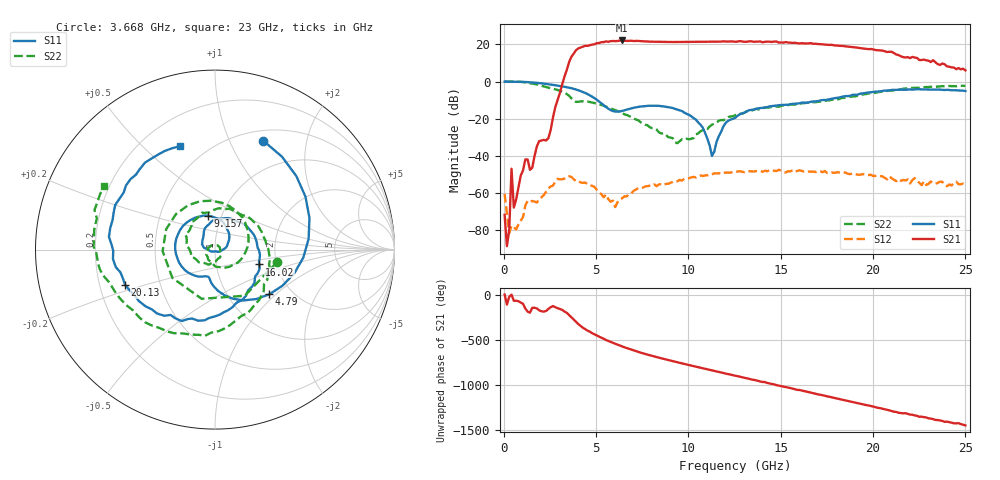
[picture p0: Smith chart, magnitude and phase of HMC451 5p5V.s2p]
!Hittite Microwave Corporation
!20 Alpha Road
!Chelmsford, MA 01824
!Tel: 978-250-3343
!Fax: 978-250-3373
!Device: HMC451, 5-20 GHz, Driver Amplifier Die
!Misc: Vcc = 5.5V, room. Die measured in housing that includes two K connectors, not de-embedded.
# MHZ S MA R 50
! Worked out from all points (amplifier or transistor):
!   201 points, 50 MHz to 25 GHz, reference 50 ohm
!   highest |S21| = 22.1 dB at 6.412 GHz (marker M1)
!   |S21| within 3 dB of that: 4.382 GHz to 18.4 GHz (14.02 GHz wide, 123 % of centre)
!   unconditionally stable (mu >= 1): start of sweep to end of sweep
!   at 4.167 GHz: K = 20.07, MAG = 20.3 dB, |S12| = -54.3 dB
!   at 12.53 GHz: K = 10.97, MAG = 21.5 dB, |S12| = -48.4 dB
!   at 25 GHz: K = 41.70, MAG = 11.5 dB, |S12| = -55.3 dB
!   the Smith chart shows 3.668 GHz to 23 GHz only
!   S11 on the Smith chart (normalised r, x): 3.668 GHz: 0.62, +1.34; 4.79 GHz: 1.54, -0.91; 9.157 GHz: 0.86, +0.34; 16.02 GHz: 1.63, -0.29; 20.13 GHz: 0.31, -0.17; 23 GHz: 0.36, +0.66
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50  0.997 -3.6  0.0002606 7.4  0.0009547 8.9  0.994 -3.9
3168.75  0.743 112.1  0.846 -162.6  0.002345 96.6  0.537 98.1
3667.75  0.664 66.2  4.674 114.0  0.002701 56.2  0.354 -11.0
3917.25  0.611 42.2  6.99 64.6  0.002066 31.6  0.284 -105.1
4291.5  0.525 6.5  8.704 -1.1  0.001883 19.2  0.295 157.3
4790.5  0.392 -39.4  9.864 -61.4  0.001564 5.8  0.273 94.1
5414.25  0.232 -85.4  11.52 -122.5  0.0007724 -4.3  0.224 40.7
5913.25  0.161 -101.5  12.33 -168.3  0.000627 14.8  0.181 3.8
6412.25  0.162 -112.5  12.76 151.7  0.0007245 51.9  0.145 -30.3
7285.5  0.208 -153.2  12.39 91.6  0.001365 42.7  0.091 -90.8
8408.25  0.222 143.8  11.68 26.9  0.00172 27.3  0.043 -165.6
9156.75  0.194 101.8  11.58 -11.5  0.002019 22.2  0.03 125.5
10778.5  0.058 8.4  11.76 -90.1  0.002875 3.7  0.049 -52.4
12525  0.105 126.8  11.77 -172.8  0.003784 -28.8  0.123 -157.3
14396.25  0.214 42.2  11.81 100.7  0.004109 -67.7  0.201 119.6
16018  0.261 -18.5  10.62 28.6  0.004087 -95.8  0.25 49.1
16766.5  0.292 -45.2  10.38 -7.6  0.003787 -108.1  0.278 21.2
18388.25  0.398 -98.3  9.058 -81.4  0.003525 -141.1  0.363 -43.9
20134.75  0.538 -158.6  7.058 -161.8  0.002915 -174.4  0.5 -110.8
20883.25  0.577 177.2  6.337 162.7  0.00284 167.2  0.566 -137.8
23004  0.608 108.5  3.648 74.3  0.001774 144.2  0.711 150.0
25000  0.558 49.2  2.006 -4.6  0.001717 113.9  0.761 88.1
